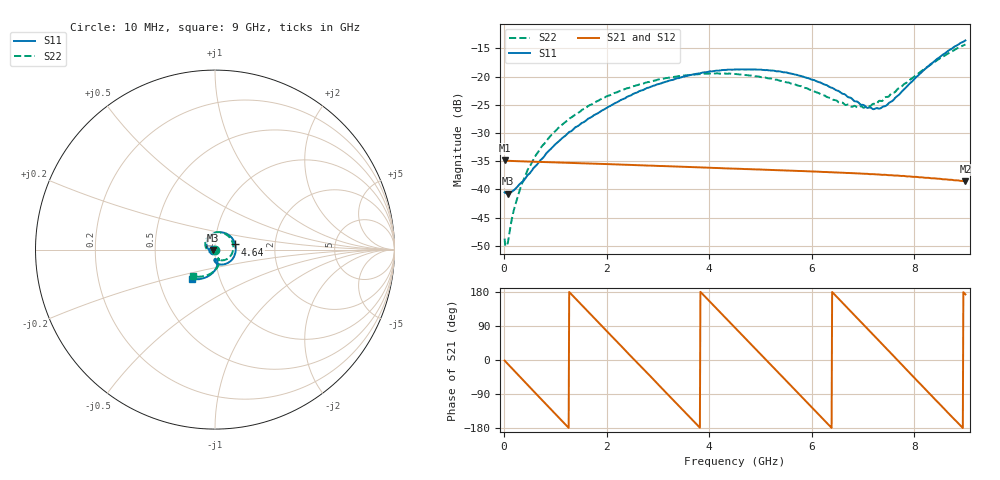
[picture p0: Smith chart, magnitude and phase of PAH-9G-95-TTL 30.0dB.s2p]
! MTS Systemtechnik GmbH
! S-Parameters
! Model: PAH-9G/95-TTL
! Attenuation Step: 30.0dB
#  HZ  S  DB  R  50.00
! Rohde & Schwarz Vector Network Analyzer
! Rohde-Schwarz,ZNB20-2Port,1334333062101652,3.45
! Created: UTC 1/26/2024, 7:20:46 AM
! freq[Hz]  db:S11  ang:S11  db:S21  ang:S21  db:S12  ang:S12  db:S22  ang:S22
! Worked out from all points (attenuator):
!   900 points, 10 MHz to 9 GHz, reference 50 ohm
!   highest |S21| = -34.85 dB at 10 MHz (marker M1); lowest = -38.5 dB at 9 GHz (marker M2)
!   lowest |S11| = -40.7 dB at 80 MHz (marker M3), VSWR 1.02, Z = 49.1 - j0.134 ohm
!   |S11| at or under -10 dB: start of sweep to end of sweep
!   |S22| runs from -50.0 to -14.3 dB; largest |S21 - S12| = 0.00052
!   S11 on the Smith chart (normalised r, x): 10 MHz: 0.98, -0.00; 4.64 GHz: 1.25, +0.07; 9 GHz: 0.73, -0.25
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1e7  -40.51 -165.4  -34.85 -1.4  -34.86 -1.4  -48.71 -138.6
5e7  -40.66 -172.8  -34.89 -7.3  -34.91 -7.3  -49.97 -148.4
8e7  -40.75 -171.4  -34.91 -11.7  -34.93 -11.7  -49.10 -139.2
1.8e8  -40.20 -165.4  -34.96 -26.1  -34.98 -26.1  -44.01 -124.2
3.1e8  -38.99 -158.9  -35.00 -44.6  -35.02 -44.6  -39.96 -124.0
4.5e8  -37.56 -155.7  -35.04 -64.5  -35.06 -64.5  -36.72 -129.0
5.9e8  -36.04 -155.5  -35.08 -84.4  -35.10 -84.3  -34.33 -135.7
9.6e8  -32.38 -165.0  -35.19 -136.8  -35.21 -136.7  -30.01 -156.6
1.51e9  -28.23 174.2  -35.36 145.6  -35.38 145.8  -25.96 170.7
2.14e9  -24.82 145.0  -35.54 57.0  -35.56 57.1  -22.95 135.7
3.01e9  -21.31 102.3  -35.82 -65.1  -35.85 -65.0  -20.51 90.3
3.76e9  -19.48 62.3  -36.08 -170.2  -36.10 -169.8  -19.59 53.2
4.51e9  -18.74 21.4  -36.31 84.9  -36.34 85.2  -19.53 16.9
4.64e9  -18.71 14.3  -36.35 66.6  -36.39 67.0  -19.65 10.7
5.38e9  -19.08 -27.6  -36.60 -37.4  -36.62 -36.4  -20.72 -24.8
6.01e9  -20.54 -62.1  -36.80 -125.9  -36.83 -124.7  -22.43 -52.3
6.54e9  -22.62 -85.9  -37.01 159.7  -37.04 160.9  -24.61 -68.0
6.9e9  -24.48 -93.3  -37.17 109.0  -37.19 110.3  -25.50 -70.5
7.21e9  -25.76 -88.6  -37.29 65.4  -37.35 66.4  -24.80 -67.9
7.51e9  -24.64 -80.2  -37.46 23.2  -37.48 24.3  -23.47 -69.4
8.26e9  -18.29 -92.7  -37.92 -82.9  -37.99 -81.4  -18.26 -93.4
9e9  -13.58 -128.4  -38.53 173.2  -38.61 174.9  -14.29 -130.0
